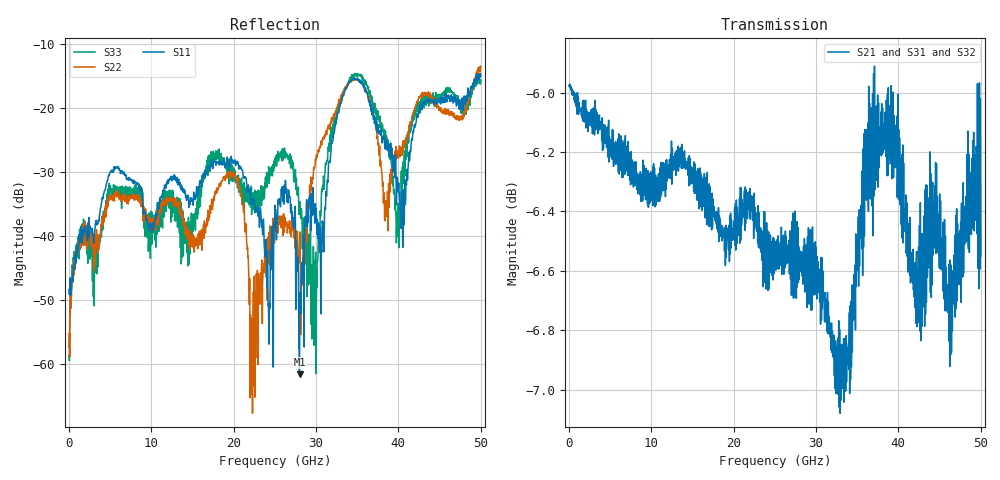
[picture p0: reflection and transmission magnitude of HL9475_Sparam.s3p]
! 1/15/2020 9:52:29 AM
! H:\PRODUCTION_DATA\9475\9475-PROTO1-01-15-2020.S3P
! CHANNEL.1
! TR.MEASUREMENT
! CORRECTED.DATA
# GHZ S RI R 50.0
! FREQ.GHZ  S11RE  S11IM  S12RE  S12IM  S13RE  S13IM
!  S21RE  S21IM  S22RE  S22IM  S23RE  S23IM
!  S31RE  S31IM  S32RE  S32IM  S33RE  S33IM
!; PortSelection: Port_123
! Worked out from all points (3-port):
!   1429 points, 35 MHz to 50.02 GHz, reference 50 ohm
!   strongest paths, dB at 35 MHz, 12.53 GHz, 25.02 GHz, 37.52 GHz, 50.02 GHz:
!     S21: -6.0, -6.2, -6.5, -6.3, -6.5
!     S31: -6.0, -6.3, -6.6, -6.3, -6.5
!     S32: -6.1, -6.5, -6.6, -6.3, -7.2
!   lowest |S11| = -61.5 dB at 28 GHz (marker M1), VSWR 1.00, Z = 49.9 + j0.036 ohm
!   |S11| at or under -10 dB: start of sweep to end of sweep
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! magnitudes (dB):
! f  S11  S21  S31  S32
! 35 MHz  -48.3  -6.0  -6.0  -6.1
! 5.67 GHz  -29.3  -6.2  -6.3  -6.3
! 19.98 GHz  -28.7  -6.5  -6.5  -6.5
! 22.23 GHz  -34.5  -6.4  -6.4  -6.4
! 25.02 GHz  -35.2  -6.5  -6.6  -6.6
! 28 GHz  -61.5  -6.6  -6.6  -6.5
! 29.86 GHz  -38.0  -6.7  -6.7  -6.6
! 34.12 GHz  -15.9  -6.7  -6.9  -6.7
! 39.94 GHz  -32.3  -6.0  -6.6  -6.4
! 50.02 GHz  -15.0  -6.5  -6.5  -7.2
